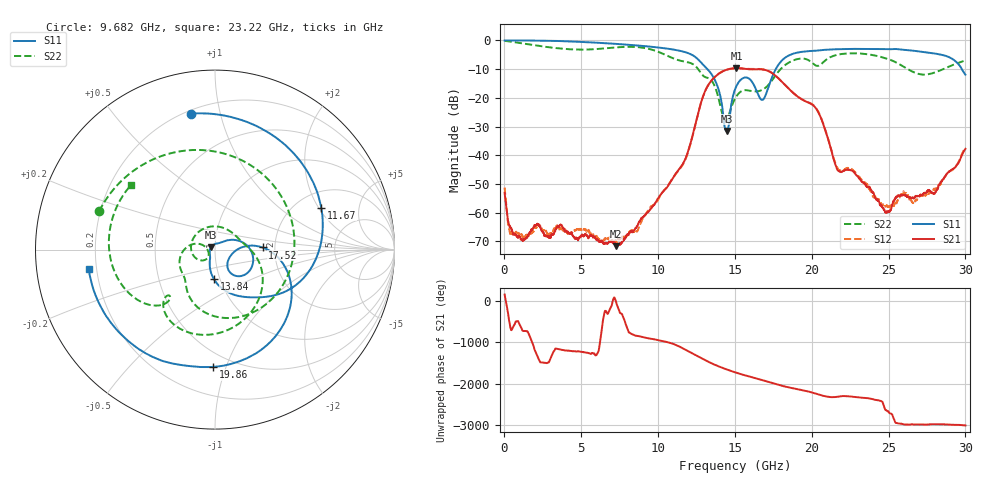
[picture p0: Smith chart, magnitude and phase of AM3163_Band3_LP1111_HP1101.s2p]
!Agilent Technologies,E8364B,MY43040894,A.07.50.67
!Agilent E8364B: A.07.50.67
!Date: Thursday, August 20, 2020 12:17:41
!Correction: S11(Full 2 Port(1,2))
!S21(Full 2 Port(1,2))
!S12(Full 2 Port(1,2))
!S22(Full 2 Port(1,2))
!S2P File: Measurements: S11, S21, S12, S22:
# Hz S  dB  R 50
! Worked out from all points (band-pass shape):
!   3201 points, 10 MHz to 30 GHz, reference 50 ohm
!   highest |S21| = -9.64 dB at 15.1 GHz (marker M1); lowest = -71.6 dB at 7.254 GHz (marker M2)
!   |S21| within 3 dB of the highest: 13.71 GHz to 17.72 GHz (4.009 GHz wide, 25.5 % of centre)
!   lowest |S11| = -31.5 dB at 14.45 GHz (marker M3), VSWR 1.05, Z = 47.8 + j1.43 ohm
!   |S11| at or under -10 dB: 13.21 GHz to 17.66 GHz (4.45 GHz wide, 28.8 % of centre); 29.77 GHz to end of sweep
!   |S22| runs from -28.2 to -0.2 dB; largest |S21 - S12| = 0.0084
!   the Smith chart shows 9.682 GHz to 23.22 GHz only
!   S11 on the Smith chart (normalised r, x): 9.682 GHz: 0.22, +0.81; 11.67 GHz: 2.69, +2.11; 13.84 GHz: 0.94, -0.32; 17.52 GHz: 1.72, +0.04; 19.86 GHz: 0.40, -0.90; 23.22 GHz: 0.17, -0.07
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1e7  -0.02 -1.9  -53.02 150.9  -51.22 129.4  -0.16 -5.3
1.256459e9  -0.01 -33.5  -69.07 -9.9  -68.75 -141.3  -1.12 -82.4
2.671612e9  -0.10 -71.0  -68.20 -57.9  -66.33 -72.2  -2.22 -162.5
5.014581e9  -0.53 -130.9  -67.82 -152.1  -66.04 -147.9  -3.20 75.1
7.254459e9  -1.20 171.8  -71.65 -14.4  -69.72 172.4  -2.43 -48.4
8.360341e9  -1.64 141.1  -66.64 -94.9  -66.30 -100.7  -2.24 -112.3
9.681775e9  -2.27 100.2  -57.52 154.8  -57.30 149.9  -3.35 161.7
1.000979e10  -2.46 88.9  -54.87 130.3  -55.35 130.0  -3.96 136.9
1.166861e10  -3.93 21.5  -42.39 -77.7  -42.74 -77.8  -7.31 -18.2
1.384289e10  -15.64 -92.0  -12.03 -127.4  -11.95 -126.7  -18.36 164.7
1.445206e10  -31.48 146.0  -10.21 145.3  -10.22 145.5  -27.92 -151.6
1.5005e10  -17.07 20.8  -9.65 75.0  -9.73 75.8  -20.30 -141.2
1.509872e10  -15.88 14.1  -9.64 63.8  -9.71 64.7  -19.47 -147.2
1.646701e10  -18.30 -54.9  -10.04 -80.8  -9.91 -80.7  -17.72 65.1
1.751666e10  -11.53 2.6  -11.74 164.2  -11.72 164.4  -13.12 -6.8
1.985963e10  -3.69 -90.8  -21.82 -36.7  -21.70 -36.0  -7.11 -130.1
2.000958e10  -3.64 -95.0  -22.27 -51.9  -22.13 -51.2  -7.74 -134.5
2.168715e10  -3.05 -136.5  -45.19 -154.7  -44.60 -149.9  -4.97 -163.2
2.322413e10  -2.95 -171.3  -48.93 -177.2  -48.49 -176.6  -4.58 142.1
2.500479e10  -3.04 145.7  -59.58 -153.5  -57.68 -116.7  -6.55 67.9
2.740399e10  -4.13 78.0  -53.18 -108.2  -53.96 -104.0  -11.90 -88.2
3e10  -11.91 -27.6  -37.75 -127.7  -37.32 -126.5  -6.96 130.5
